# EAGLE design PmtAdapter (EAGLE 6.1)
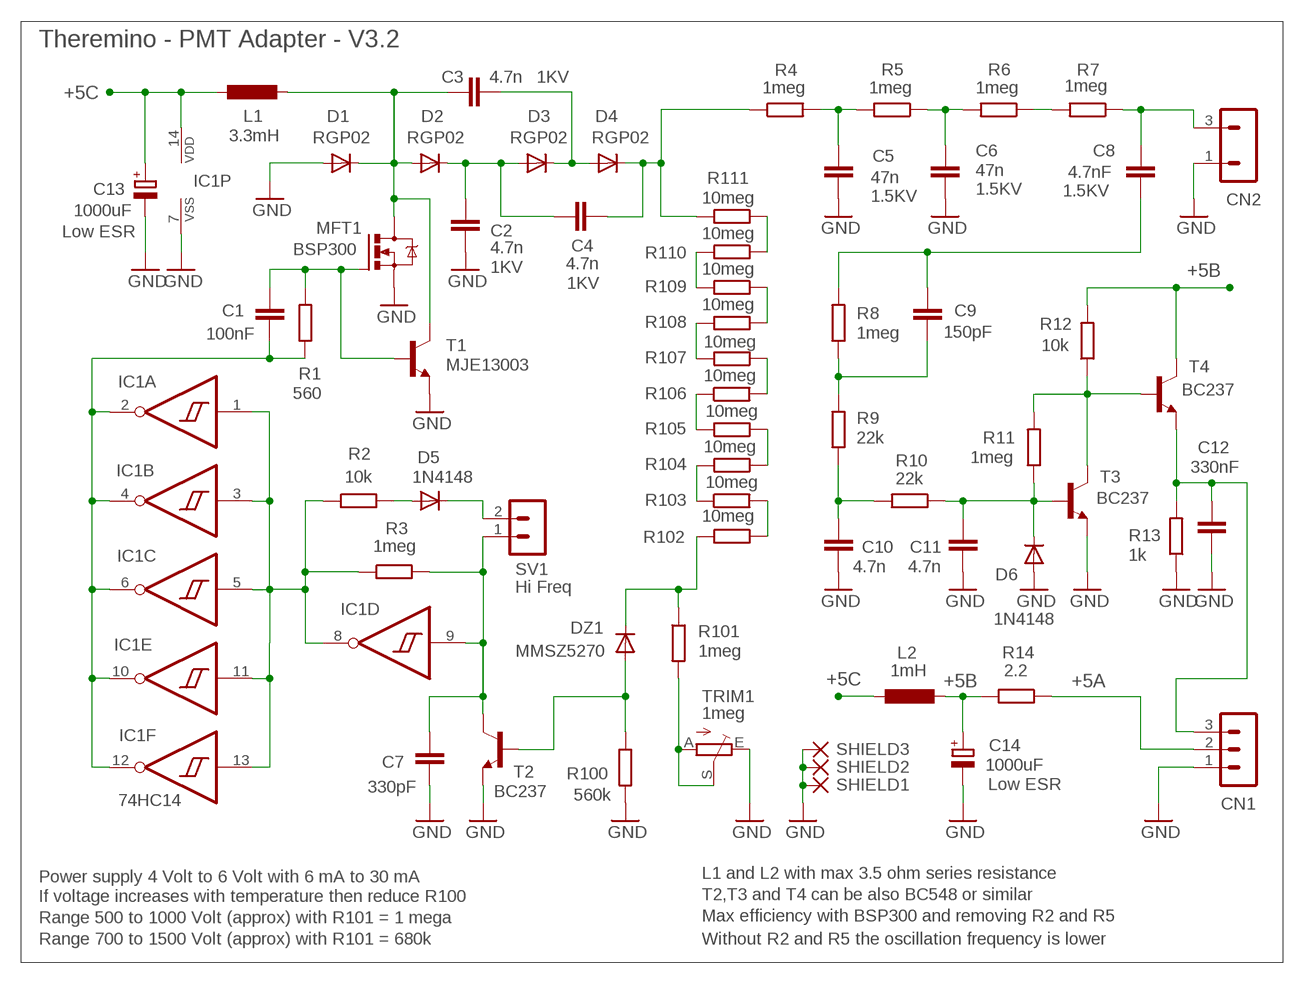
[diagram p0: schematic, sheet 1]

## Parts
C1  100nF  C-EU050-024X044  [C050-024X044]
C2  4.7n  C5/2.5  [C5B2.5]
C3  4.7n  C5/2.5  [C5B2.5]
C4  4.7n  C5/2.5  [C5B2.5]
C5  47n  C-EUC2220K  [C2220K]
C6  47n  C-EUC2220K  [C2220K]
C7  330pF  C-EU025-024X044  [C025-024X044]
C8  4.7nF  C-EU075-032X103  [C075-032X103]
C9  150pF  C-EU050-024X044  [C050-024X044]
C10  4.7n  C-EU050-024X044  [C050-024X044]
C11  4.7n  C-EU050-024X044  [C050-024X044]
C12  330nF  C-EU050-024X044  [C050-024X044]
C13  1000uF  CPOL-EUE5-10.5  [E5-10,5]
C14  1000uF  CPOL-EUE5-10.5  [E5-10,5]
CN1  MA03-1N  [MA03-1]
CN2  MA03-1-2  [MA03-1-2]
D1  RGP02  DIODE-DO34-7  [DO34-7]
D2  RGP02  DIODE-DO34-7  [DO34-7]
D3  RGP02  DIODE-DO34-7  [DO34-7]
D4  RGP02  DIODE-DO34-7  [DO34-7]
D5  1N4148  DIODE-DO34-7  [DO34-7]
D6  1N4148  DIODE-D-5  [D-5]
DZ1  MMSZ5270  DIODE-DO34-7  [DO34-7]
IC1  74HC14  40106N  [DIL14]
L1  3.3mH  INDUCTORL_VERT_508  [L_VERT_508]
L2  1mH  INDUCTORL_VERT_508  [L_VERT_508]
MFT1  BSP300  [SOT223]
R1  560  R-EU_0204/7  [0204/7]
R2  10k  R-EU_0204/7  [0204/7]
R3  1meg  R-EU_0204/7  [0204/7]
R4  1meg  R-EU_0204/7  [0204/7]
R5  1meg  R-EU_R1206  [R1206]
R6  1meg  R-EU_R1206  [R1206]
R7  1meg  R-EU_R1206  [R1206]
R8  1meg  R-EU_0204/7  [0204/7]
R9  22k  R-EU_0204/7  [0204/7]
R10  22k  R-EU_0204/7  [0204/7]
R11  1meg  R-EU_0204/7  [0204/7]
R12  10k  R-EU_0204/7  [0204/7]
R13  1k  R-EU_0204/7  [0204/7]
R14  2.2  R-EU_R1206  [R1206]
R100  560k  R-EU_0204/7  [0204/7]
R101  1meg  R-EU_0204/7  [0204/7]
R102  10meg  R-EU_R1206  [R1206]
R103  10meg  R-EU_R1206  [R1206]
R104  10meg  R-EU_R1206  [R1206]
R105  10meg  R-EU_R1206  [R1206]
R106  10meg  R-EU_R1206  [R1206]
R107  10meg  R-EU_R1206  [R1206]
R108  10meg  R-EU_R1206  [R1206]
R109  10meg  R-EU_R1206  [R1206]
R110  10meg  R-EU_R1206  [R1206]
R111  10meg  R-EU_R1206  [R1206]
SHIELD1  WIREPAD2,15/1,0  [2,15/1,0]
SHIELD2  WIREPAD2,15/1,0  [2,15/1,0]
SHIELD3  WIREPAD2,15/1,0  [2,15/1,0]
SV1  Hi Freq  MA02-1L2  [MA02-1_L2]
T1  MJE13003  -NPN-TO92-BCE  [TO92-BCE]
T2  BC237  -NPN-TO92-CBE  [TO92-CBE]
T3  BC237  -NPN-TO92-CBE  [TO92-CBE]
T4  BC237  -NPN-TO92-CBE  [TO92-CBE]
TRIM1  1meg  TRIM_EU-PT10  [PT-10]

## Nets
+5A: CN1.2 R14.1
+5B: C14.+ L2.+ R12.2 R14.2 T4.C
+5C: C13.+ IC1.14(P:VDD) L1.- L2.-
GND: C2.2 C5.2 C6.2 C7.2 C10.1 C11.1 C12.1 C13.- C14.- CN1.1 CN2.1 D1.A D6.A IC1.7(P:VSS) MFT1.3(S) R13.1 R100.2 SHIELD1.1(P) SHIELD2.1(P) SHIELD3.1(P) T1.E T2.E T3.E TRIM1.E
N$1: C1.2 IC1.2(A:O) IC1.4(B:O) IC1.6(C:O) IC1.10(E:O) IC1.12(F:O) R1.1
N$2: D5.A R2.2
N$3: R11.2 R12.1 T3.C T4.B
N$4: DZ1.A R100.1 T2.B
N$5: C1.1 MFT1.1(G) R1.2 T1.B
N$6: C9.2 R8.1 R9.2
N$7: IC1.1(A:I) IC1.3(B:I) IC1.5(C:I) IC1.8(D:O) IC1.11(E:I) IC1.13(F:I) R2.1 R3.1
N$8: C8.2 CN2.3 R7.1
N$9: C2.1 C4.2 D2.C D3.A
N$10: C3.2 D3.C D4.A
N$11: R101.2 TRIM1.A TRIM1.S
N$12: C4.1 D4.C R4.1 R111.2
N$13: C5.1 R4.2 R5.2
N$14: C7.1 IC1.9(D:I) R3.2 SV1.1 T2.C
N$15: C6.1 R5.1 R6.2
N$16: C3.1 D1.C D2.A L1.+ MFT1.2(D) MFT1.4(D) T1.C
N$17: C10.2 R9.1 R10.2
N$18: C11.2 D6.C R10.1 R11.1 T3.B
N$19: C8.1 C9.1 R8.2
N$20: R107.2 R108.2
N$21: R108.1 R109.1
N$22: R109.2 R110.2
N$23: R110.1 R111.1
N$24: R104.1 R105.1
N$25: R105.2 R106.1
N$26: R103.1 R104.2
N$27: R106.2 R107.1
N$28: R102.1 R103.2
N$29: DZ1.C R101.1 R102.2
N$30: R6.1 R7.2
N$31: D5.C SV1.2
N$32: C12.2 CN1.3 R13.2 T4.E

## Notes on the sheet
- Theremino - PMT Adapter - V3.2
- Power supply 4 Volt to 6 Volt with 6 mA to 30 mA | L1 and L2 with max 3.5 ohm series resistance
- If voltage increases with temperature then reduce R100 | T2,T3 and T4 can be also BC548 or similar
- Range 500 to 1000 Volt (approx) with R101 = 1 mega | Max efficiency with BSP300 and removing R2 and R5
- Range 700 to 1500 Volt (approx) with R101 = 680k | Without R2 and R5 the oscillation frequency is lower

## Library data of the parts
C1 C7 C9-C12 = 00-LIVIO:C-EU: CAPACITOR, European symbol
C2-C4 = 00-LIVIO:C: CAPACITOR; VOLTAGE: 1KV
C5 C6 C8 = 00-LIVIO:C-EU: CAPACITOR, European symbol; VOLTAGE: 1.5KV
C13 C14 = 00-LIVIO:CPOL-EU: POLARIZED CAPACITOR, European symbol; 1: Low ESR
CN1 = 03-con-lstb-M:MA03-1: PIN HEADER
CN2 = 03-con-lstb-M:MA03-1-2; 1: PMT+; 2: PMT-
D1-D6 DZ1 = 00-LIVIO:DIODE-: DIODE
IC1 = 40xx:40106: Hex SCHMITT TRIGGER
L1 L2 = 00-LIVIO:INDUCTOR
MFT1 = 00-LIVIO:BSP300: MOSFET 800V
R1-R14 R100-R111 = 00-LIVIO:R-EU_: RESISTOR, European symbol
SHIELD1-SHIELD3 = 00-LIVIO:WIREPAD: Wire PAD connect wire on PCB
SV1 = 03-con-lstb-M:MA02-1: PIN HEADER
T1-T4 = 00-LIVIO:*-NPN-: NPN Transistror
TRIM1 = 00-LIVIO:TRIM_EU-: POTENTIOMETER

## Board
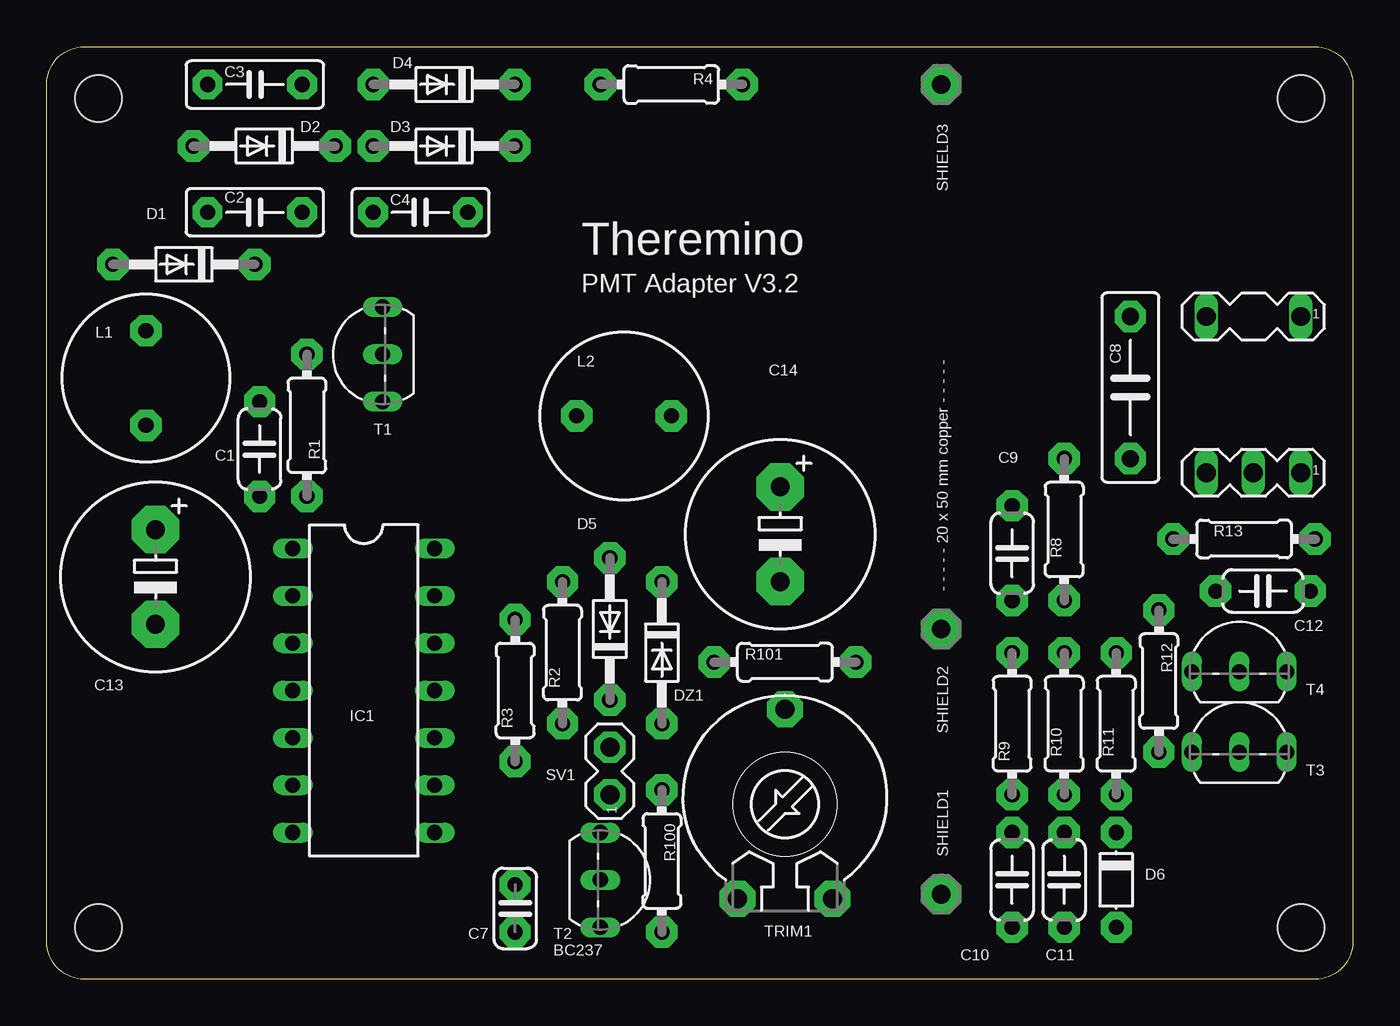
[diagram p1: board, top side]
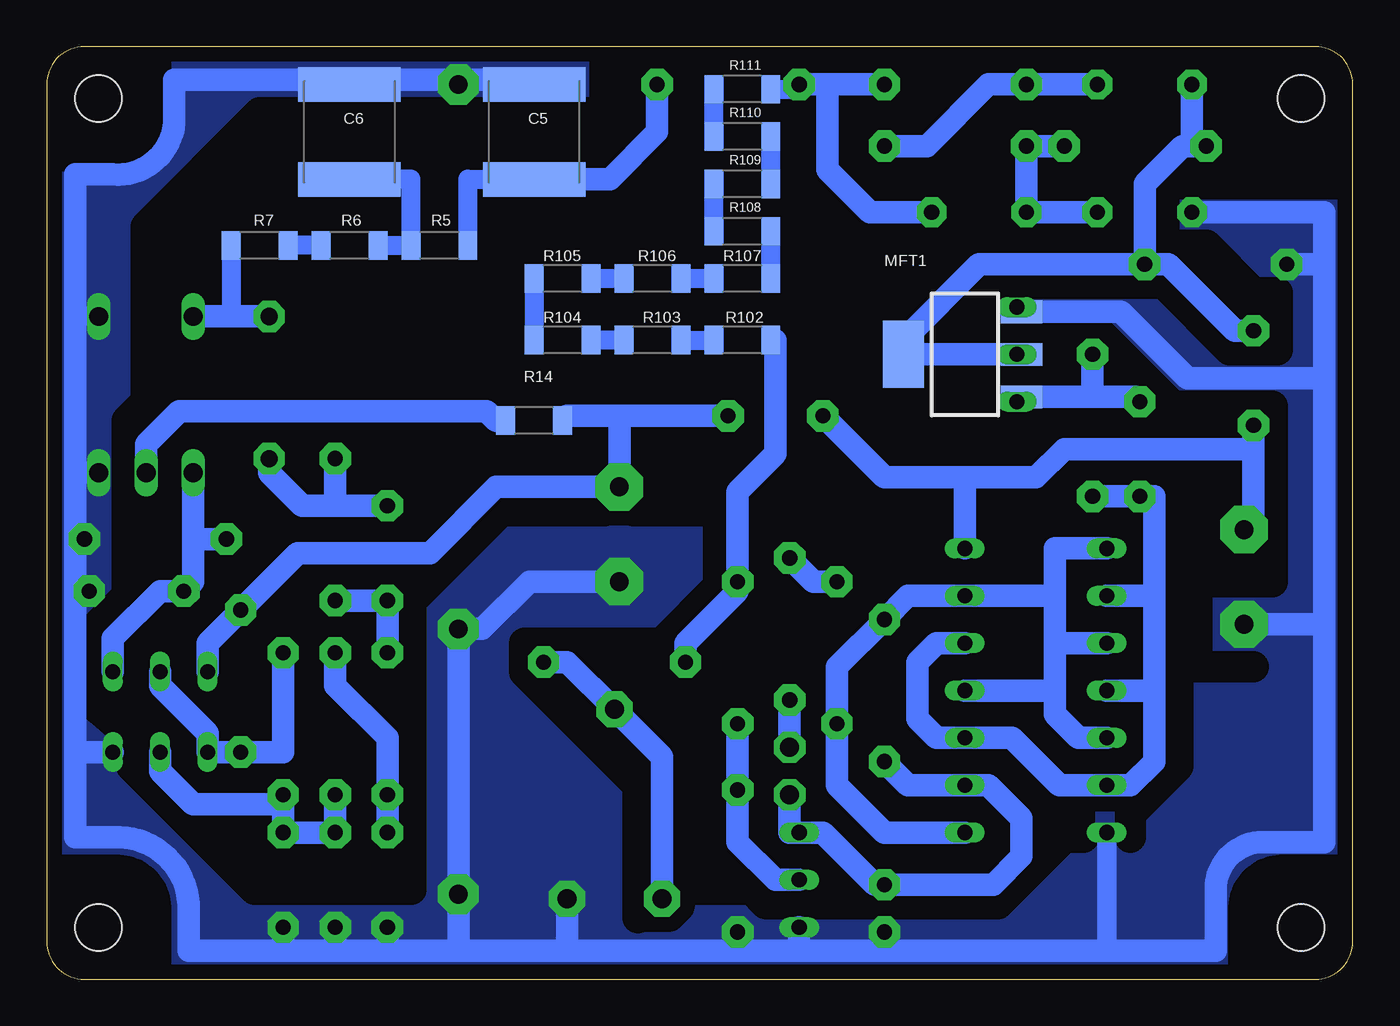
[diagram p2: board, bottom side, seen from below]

Size 70.1 x 50.04 mm. Coordinates in mm from the lower left corner, seen from the top.
Outline: 2.03,0 arc-90 0,2.03 0,48.01 arc-90 2.03,50.04 68.07,50.04 arc-90 70.1,48.01 70.1,2.03 arc-90 68.07,0 2.03,0
Copper layers (1*16): Top 0.035mm / dielectric 1.5mm / Bottom 0.035mm
Design rules: minimum track width 10mil, minimum drill 27mil, track to track 27mil, track to pad 27mil, pad to pad 27mil, via to via 27mil, smd to smd 27mil, copper to edge 27mil, drill to drill 8mil, minimum pad ring 5mil, minimum via ring 8mil, stop-mask expansion 4mil, vias tented up to drill 0mil, thermal gap 41mil
Holes 2.5 mm at 2.79,47.24 67.31,47.24 67.31,2.79 2.79,2.79
bRestrict: 59 lines

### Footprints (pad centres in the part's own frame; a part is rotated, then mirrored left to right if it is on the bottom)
C050-024X044 = drill 0.813 pad 1.676 octagon: 1 -2.54,0; 2 2.54,0
C5B2.5 = drill 0.813 pad 1.6 octagon: 1 -2.54,0; 2 2.54,0
C2220K = smd 1.85 x 5.5: 1 -2.55,0; 2 2.55,0
C025-024X044 = drill 0.813 pad 1.676 octagon: 1 -1.27,0; 2 1.27,0
C075-032X103 = drill 0.914 pad 1.676 octagon: 1 -3.81,0; 2 3.81,0
E5-10,5 = drill 1.016 pad 2.54 octagon: + -2.54,0; - 2.54,0
MA03-1 = drill 1.016 long: 1 -2.54,0; 2 0,0; 3 2.54,0
MA03-1-2 = drill 1.016 long: 1 -2.54,0; 3 2.54,0
DO34-7 = drill 0.813 pad 1.676 octagon: A 3.81,0; C -3.81,0
D-5 = drill 0.813 pad 1.676 octagon: A 2.54,0; C -2.54,0
DIL14 = drill 0.813 long: 1 -7.62,-3.81; 2 -5.08,-3.81; 3 -2.54,-3.81; 4 0,-3.81; 5 2.54,-3.81; 6 5.08,-3.81; 7 7.62,-3.81; 8 7.62,3.81; 9 5.08,3.81; 10 2.54,3.81; 11 0,3.81; 12 -2.54,3.81; 13 -5.08,3.81; 14 -7.62,3.81
L_VERT_508 = drill 0.813 pad 1.676 octagon: + -2.54,0; - 2.54,0
SOT223 = smd 1.219 x 2.235: 1 -2.286,-3.048; 2 0,-3.048; 3 2.286,-3.048 | smd 3.6 x 2.2: 4 0,3.302
0204/7 = drill 0.813 pad 1.676 octagon: 1 -3.81,0; 2 3.81,0
R1206 = smd 1.016 x 1.524: 1 -1.524,0; 2 1.524,0
2,15/1,0 = drill 1.016 pad 2.159 octagon: 1 0,0
MA02-1_L2 = drill 1.016 pad 1.676 octagon: 1 -1.27,0; 2 1.27,0
TO92-BCE = drill 0.813 long: B -2.54,0; C 0,0; E 2.54,0
TO92-CBE = drill 0.813 long: B 0,0; C -2.54,0; E 2.54,0
PT-10 = drill 1.016 pad 1.93 octagon: A -2.54,-5.08; E 2.54,-5.08; S 0,5.08

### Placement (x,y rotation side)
C1  11.43,28.45 270 top
C2  11.18,41.15 180 top
C3  11.18,48.01 0 top
C4  20.07,41.15 180 top
C5  43.94,45.47 90 bottom
C6  53.85,45.47 90 bottom
C7  25.15,3.81 270 top
C8  58.17,31.75 90 top
C9  51.82,22.86 270 top
C10  51.82,5.33 90 top
C11  54.61,5.33 90 top
C12  65.28,20.83 180 top
C13  5.84,21.59 270 top
C14  39.37,23.88 270 top
CN1  64.77,27.18 180 top
CN2  64.77,35.56 180 top
D1  7.37,38.35 180 top
D2  11.68,44.7 180 top
D3  21.34,44.7 180 top
D4  21.34,48.01 180 top
D5  30.23,18.8 90 top
D6  57.4,5.33 270 top
DZ1  33.02,17.53 270 top
IC1  17.02,15.49 270 top
L1  5.33,32.26 270 top
L2  30.99,30.23 180 top
MFT1  20.83,33.53 90 bottom
R1  13.97,29.72 90 top
R2  27.69,17.53 90 top
R3  25.15,15.49 270 top
R4  33.53,48.01 0 top
R5  49.02,39.37 0 bottom
R6  53.85,39.37 0 bottom
R7  58.67,39.37 0 bottom
R8  54.61,24.13 90 top
R9  51.82,13.72 90 top
R10  54.61,13.72 90 top
R11  57.4,13.72 90 top
R12  59.69,16 90 top
R13  64.26,23.62 180 top
R14  43.94,29.97 0 bottom
R100  33.02,6.35 270 top
R101  39.62,17.02 0 top
R102  32.77,34.29 0 bottom
R103  37.59,34.29 0 bottom
R104  42.42,34.29 0 bottom
R105  42.42,37.59 0 bottom
R106  37.59,37.59 0 bottom
R107  32.77,37.59 0 bottom
R108  32.77,40.13 0 bottom
R109  32.77,42.67 0 bottom
R110  32.77,45.21 0 bottom
R111  32.77,47.75 0 bottom
SHIELD1  48.01,4.57 0 top
SHIELD2  48.01,18.8 0 top
SHIELD3  48.01,48.01 0 top
SV1  30.23,11.18 90 top
T1  18.03,33.53 90 top
T2  29.72,5.33 270 top
T3  64.01,12.19 0 top
T4  64.01,16.51 0 top
TRIM1  39.62,9.4 0 top

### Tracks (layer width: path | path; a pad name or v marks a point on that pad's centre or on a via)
+5A
  Bottom 1.016: 45.97,29.97 R14.1
  Bottom 1.2: CN1.2 64.77,28.7 62.99,30.48 46.48,30.48 45.97,29.97
+5B
  Bottom 1.016: R14.2 42.16,30.23
  Bottom 1.2: 39.37,30.23 C14.+ 45.97,26.42 49.53,22.86 56.64,22.86 R12.2 61.47,18.03 T4.C | L2.+ 39.37,30.23 | 42.16,30.23 39.37,30.23
+5C
  Bottom 1.2: IC1.14 20.83,26.92 | 20.83,26.92 25.15,26.92 | L1.- 5.33,28.45 | 5.33,28.45 15.49,28.45 17.02,26.92 20.83,26.92 | 20.83,26.92 25.15,26.92 | 25.15,26.92 L2.- 25.15,26.92 | C13.+ 5.33,24.64 5.33,28.45
GND
  Bottom 1.016: 5.08,7.37 4.83,7.37 | 28.96,1.52 29.72,1.52 | 53.85,48.26 C6.2 | C6.2 53.85,48.01 C6.2 | C6.2 53.1,48.02 | T1.E 17.78,36.07 MFT1.3 | CN2.1 68.58,35.56 68.58,36.07
  Bottom 1.05: IC1.7 13.21,1.52
  Bottom 1.2: 68.58,12.19 68.58,7.62 66.55,7.62 arc90 62.48,4.06 62.48,1.52 57.4,1.52 | 68.58,12.19 68.58,12.45 68.58,20.83 | 68.58,23.62 68.58,27.18 | 68.58,27.18 68.58,35.56 68.58,36.07 68.58,43.18 66.55,43.18 arc-90 63.25,45.97 63.25,48.26 53.85,48.26 43.94,48.26 C5.2 | 29.72,1.52 25.15,1.52 | 25.15,1.52 29.72,1.52 | 29.72,1.52 28.96,1.52 | 28.96,1.52 29.72,1.52 | 29.72,1.52 33.02,1.52 | 33.02,1.52 29.72,1.52 | 29.72,1.52 28.96,1.52 | 28.96,1.52 29.72,1.52 | 29.72,1.52 28.96,1.52 | 28.96,1.52 29.72,1.52 | 29.72,1.52 33.02,1.52 | 33.02,1.52 42.16,1.52 | 42.16,1.52 48.01,1.52 | 1.52,20.07 1.52,24.38 | 1.52,24.38 1.52,20.07 | 1.52,20.07 1.52,19.05 | 1.52,19.05 1.52,9.4 1.52,7.87 1.52,7.37 4.83,7.37 arc-90 7.37,4.83 7.37,1.52 13.21,1.52 25.15,1.52 | 57.4,1.52 54.61,1.52 | 54.61,1.52 51.82,1.52 | 51.82,1.52 48.01,1.52 | C2.2 1.52,41.15 1.52,38.35 | 1.52,38.35 1.52,32.26 | 1.52,32.26 1.52,24.38 | 25.15,1.52 29.72,1.52 | D6.A 57.4,1.52 | C11.1 54.61,1.52 | C10.1 51.82,1.52 | CN1.1 68.58,27.18 | T2.E 29.72,1.52 | T3.E 68.58,12.19 | C7.2 25.15,1.52 | R100.2 33.02,1.52 | 29.72,1.52 33.02,1.52 | R13.1 68.58,23.62 | 48.01,1.52 SHIELD1.1 SHIELD2.1 46.74,18.8 44.2,21.34 C14.- | TRIM1.E 42.16,1.52 | 68.58,20.83 68.58,23.62 | C12.1 68.58,20.83 | 1.52,32.26 8.89,32.26 12.45,35.81 MFT1.3 | D1.A 1.52,38.35 | C13.- 1.52,19.05
  pour Bottom (isolate 0.8, no thermals): -1,-1 71.1,-1 71.1,51.04 -1,51.04
N$1
  Bottom 1.016: 10.67,15.49 IC1.4
  Bottom 1.2: 10.67,15.49 10.67,11.68 11.94,10.41 IC1.6 15.75,10.41 18.29,12.95 IC1.10 22.35,12.95 23.37,13.97 23.37,17.02 22.35,18.03 IC1.12 | IC1.4 10.67,15.49 | 10.67,15.49 10.67,20.57 | 10.67,20.57 IC1.2 | R1.1 C1.2 10.67,25.91 10.67,20.57
N$2
  Bottom 1.2: R2.2 28.96,21.34 D5.A
N$3
  Bottom 1.2: R11.2 57.4,16 57.4,12.19 R12.1 61.21,12.19 T3.C 61.47,13.21 64.01,15.75 T4.B
N$4
  Bottom 1.2: DZ1.A R100.1 33.02,7.37 30.99,5.33 T2.B
N$5
  Bottom 1.016: MFT1.1 18.03,31.24 T1.B
  Bottom 1.2: C1.1 11.68,31.24 13.97,31.24 | 13.97,31.24 R1.2 | MFT1.1 13.97,31.24
N$6
  Bottom 1.2: 51.82,18.03 C9.2 R8.1 | 51.82,18.03 R9.2 51.82,18.03
N$7
  Bottom 1.2: IC1.5 14.73,12.95 16,14.22 16,15.49 | 16,15.49 16,18.03 | 16,18.03 16,20.57 | 16,20.57 16,23.11 IC1.1 | IC1.3 16,18.03 | IC1.11 16,15.49 | 16,20.57 IC1.13 23.88,20.57 R3.1 27.69,16.76 | IC1.8 25.15,7.87 27.69,10.41 R2.1 | R2.1 27.69,16.76 | R2.1 27.69,16.76
N$8
  Bottom 1.016: C8.2 60.2,35.56 R7.1
  Bottom 1.2: CN2.3 60.2,35.56 C8.2
N$9
  Bottom 1.2: C4.2 D3.A D2.C | C4.2 C2.1 C4.2
N$10
  Bottom 1.2: C3.2 D4.A 19.56,48.01 22.86,44.7 D3.C
N$11
  Bottom 1.2: R101.2 42.16,17.02 TRIM1.S 37.08,11.94 TRIM1.A
N$12
  Bottom 1.016: R111.2 29.72,47.75
  Bottom 1.2: R4.1 28.19,48.01 | 28.19,48.01 R4.1 | D4.C R4.1 | C4.1 25.91,41.15 28.19,43.43 28.19,48.01 | 29.72,47.75 R4.1
N$13
  Bottom 1.016: C5.1 46.23,42.93 47.5,42.93 R5.2 | C5.1 43.18,42.93 | C5.1
  Bottom 1.2: R4.2 37.34,45.47 39.88,42.93 43.18,42.93
N$14
  Bottom 1.2: R3.2 23.88,10.41 IC1.9 19.56,10.41 17.78,8.64 17.78,6.6 19.3,5.08 C7.1 25.65,5.08 28.45,7.87 T2.C 30.23,7.87 SV1.1
N$15
  Bottom 1.016: C6.1 50.55,42.93 R5.1 R6.2 | C6.1 | C6.1 | C6.1
N$16
  Bottom 1.2: C3.1 8.64,44.7 D2.A 9.14,44.7 11.18,42.67 11.18,39.88 D1.C | L1.+ 6.35,34.8 9.91,38.35 | 9.91,38.35 D1.C | 9.91,38.35 D1.C | 9.91,38.35 D1.C | D1.C 20.07,38.35 24.13,34.29 24.13,33.78 MFT1.4 T1.C MFT1.2
N$17
  Bottom 1.2: C10.2 R9.1 51.82,12.95 54.61,15.75 R10.2
N$18
  Bottom 1.016: R11.1 57.4,9.4
  Bottom 1.2: R10.1 C11.2 D6.C 57.4,9.4 | T3.B 64.01,11.18 62.23,9.4 57.4,9.4 | 57.4,9.4 R11.1
N$19
  Bottom 1.2: C9.1 54.61,25.4 | 54.61,25.4 56.39,25.4 58.17,27.18 C8.1 | R8.2 54.61,25.4
N$20
  Bottom 1.016: R107.2 R108.2
N$21
  Bottom 1.016: R108.1 R109.1
N$22
  Bottom 1.016: R109.2 R110.2
N$23
  Bottom 1.016: R110.1 R111.1
N$24
  Bottom 1.016: R105.1 R104.1
N$25
  Bottom 1.016: R106.1 R105.2
N$26
  Bottom 1.016: R103.1 R104.2
N$27
  Bottom 1.016: R107.1 R106.2
N$28
  Bottom 1.016: R103.2 R102.1
N$29
  Bottom 1.016: R102.2 30.99,34.29
  Bottom 1.2: 30.99,34.29 30.99,28.19 33.02,26.16 33.02,20.83 | 33.02,20.83 35.81,18.03 R101.1 | 33.02,20.83 DZ1.C
N$30
  Bottom 1.016: R6.1 R7.2
N$31
  Bottom 1.2: SV1.2 D5.C
N$32
  Bottom 1.2: T4.E 66.55,18.29 64.01,20.83 C12.2 | C12.2 62.23,21.34 | 62.23,21.34 62.23,23.62 | 62.23,23.62 R13.2 | CN1.3 62.23,23.62 | C12.2 62.23,21.34

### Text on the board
tNames: Theremino | PMT Adapter V3.2 | - - - - - 20 x 50 mm copper - - - - -
tValues: 50x70mm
